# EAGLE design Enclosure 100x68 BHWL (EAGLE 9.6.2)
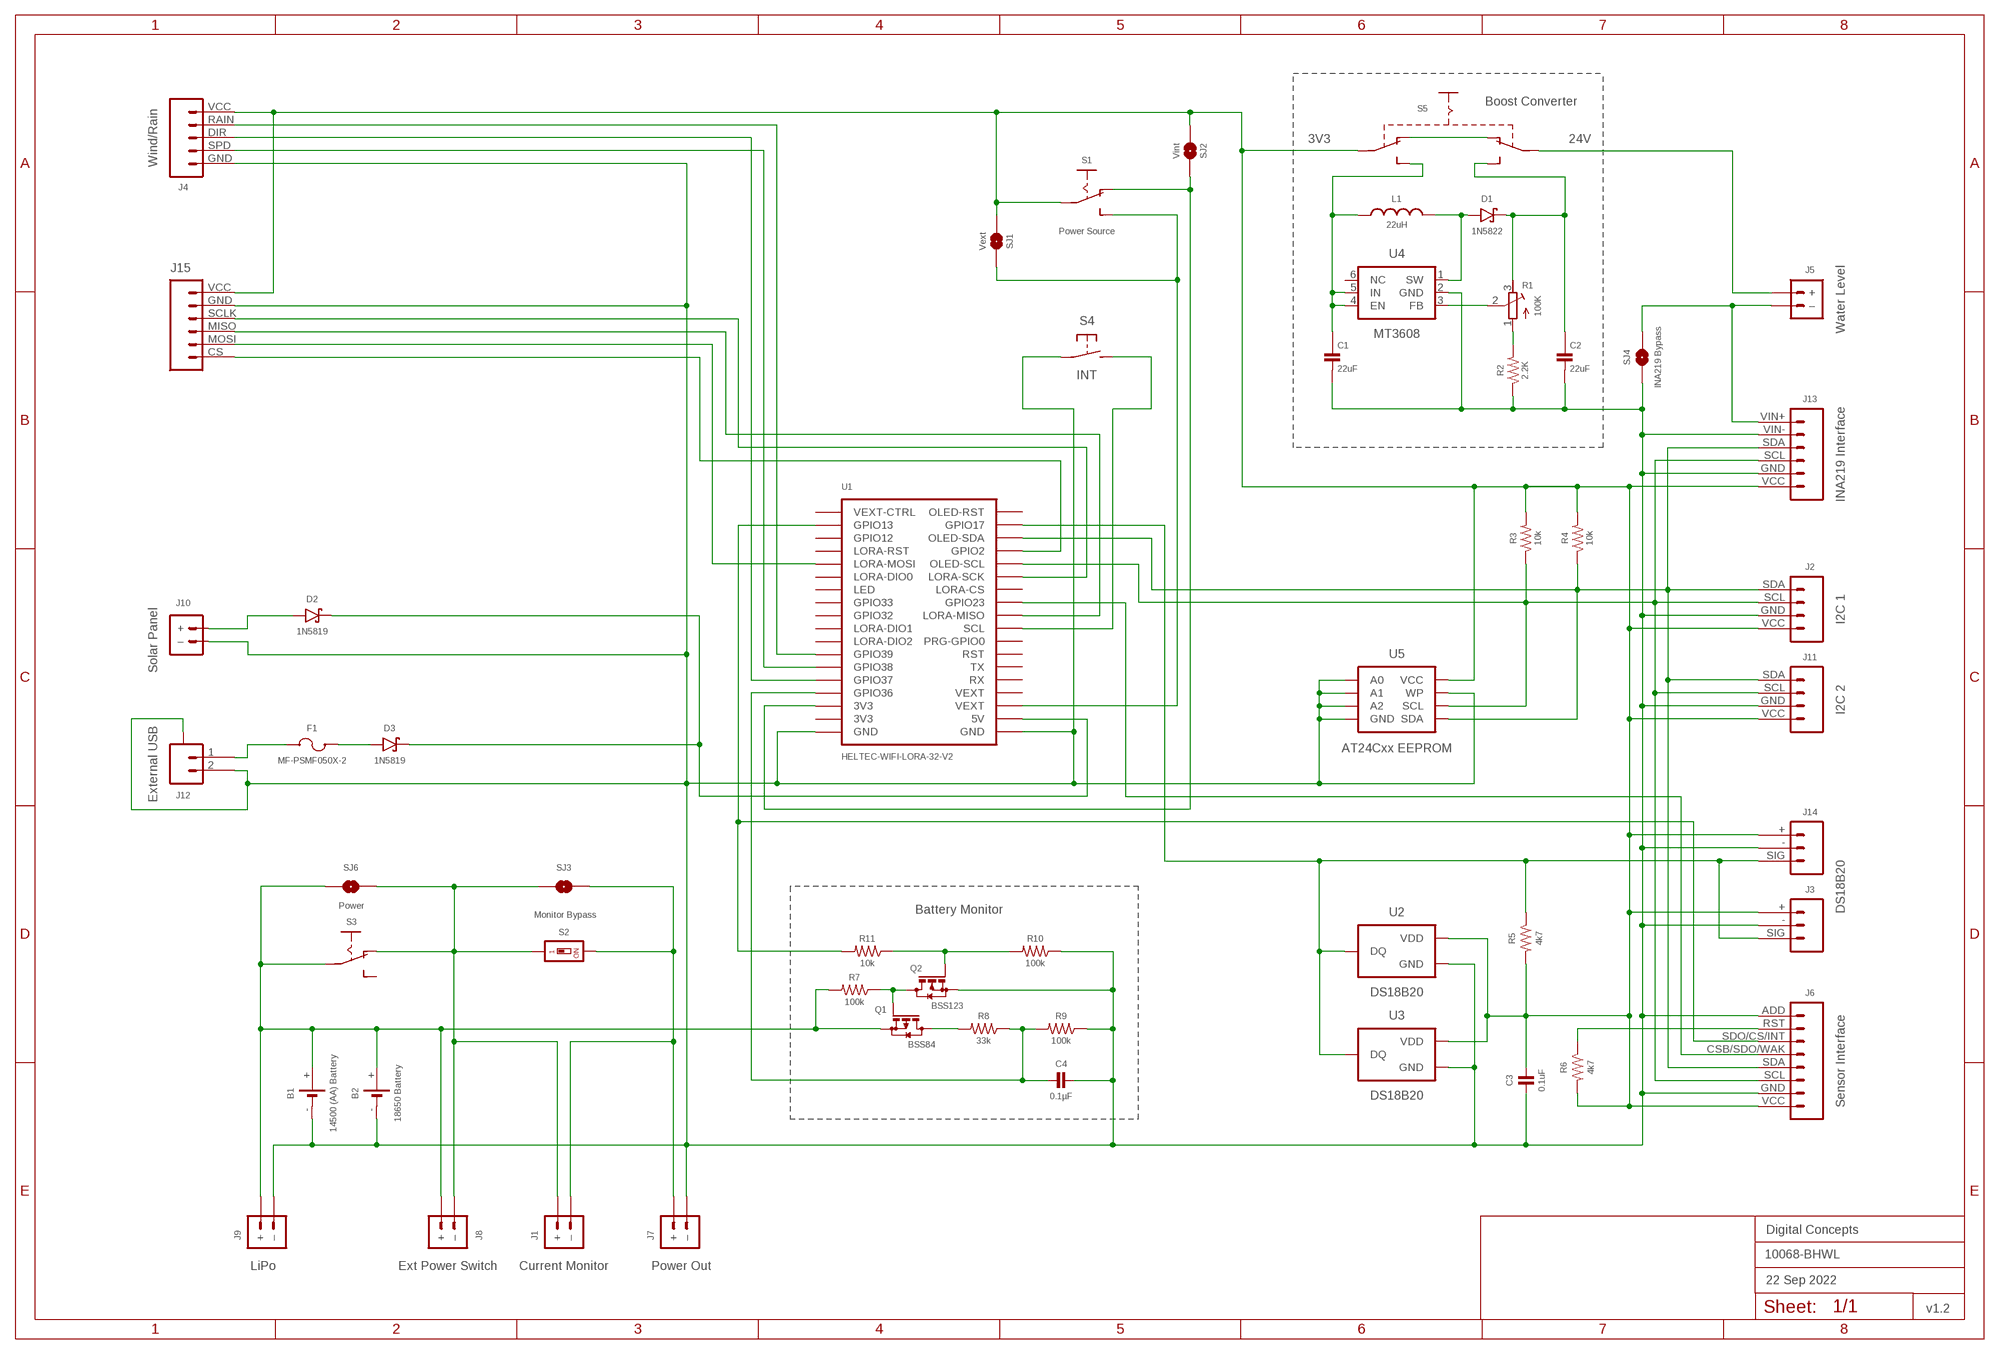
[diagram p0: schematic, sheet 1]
FRAME2 (A3L-LOC): DATE: 22 Sep 2022; OWNER: Digital Concepts; TITLE: 10068-BHWL; VERSION: v1.2

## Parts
B1  14500 (AA) Battery  BATTERY-HOLDER-14500(AA)  [BATTERY-14500]
B2  18650 Battery  BATTERY-HOLDER-18650  [BATTERY-18650]
C1  22uF  CAPACITOR-1206  [C1206]
C2  22uF  CAPACITOR-1206  [C1206]
C3  0.1uF  CAPACITOR-0805  [C0805]
C4  0.1µF  CAPACITOR-0805  [C0805]
D1  1N5822  DIODE-SCHOTTKY-1N5822  [DIODE_SMB]
D2  1N5819  1N5819-SOD-123  [SOD-123]
D3  1N5819  1N5819-SOD-123  [SOD-123]
F1  MF-PSMF050X-2  [F0805]
J1  Current Monitor  JST-PH2.0-2-HORIZONTALJST-PTH-2  [JST-PH2.0-2-HORIZONTAL]
J2  I2C 1  JST-PH2.0-4-VERTICAL-I2C  [JST-PH2.0-4-VERTICAL-I2C]
J3  DS18B20  JST-PH2.0-3-VERTICAL-DS18B20  [JST-PH2.0-3-VERTICAL-SIG]
J4  Wind/Rain  JST-PH2.0-5-DUAL-WEATHER  [JST-PH2.0-5-DUAL-WEATHER]
J5  Water Level  JST-PH2.0-2-DUAL-POWERJST-PTH-2  [JST-PH2.0-2-DUAL-POWER]
J6  Sensor Interface  HEADER-1X8-SENSOR  [CONN_08-SENSOR]
J7  Power Out  JST-GH1.25-2-HORIZONTAL-POWER  [JST-GH1.25-2-HORIZONTAL]
J8  Ext Power Switch  JST-PH2.0-2-DUAL-POWERJST-PTH-2  [JST-PH2.0-2-DUAL-POWER]
J9  LiPo  JST-PH2.0-2-HORIZONTAL-POWERJST-PTH-2  [JST-PH2.0-2-HORIZONTAL-POWER]
J10  Solar Panel  JST-PH2.0-2-VERTICAL  [JST-PH2.0-2-VERTICAL=POWER]
J11  I2C 2  JST-PH2.0-I2C-MALE-HORIZONTAL  [JST-PH2.0-4-HORIZONTAL]
J12  External USB  JST-SH1.0-2-SMD-HORIZONTAL  [JST-SH1.0-2-HORIZONTAL]
J13  INA219 Interface  INA219-I2C-MODULE  [CONN_06-INA219]
J14  JST-PH2.0-3-HORIZONTAL-DS18B20  [JST-PH2.0-DS18B20-HORIZONTAL]
J15  JST-PH2.0-6-HORIZONTAL-SPI  [JST-PH2.0-6-HORIZONTAL-SPI]
L1  22uH  INDUCTOR-CDRH104R/6D28L5038P  [CDRH104R+6D28]
Q1  BSS84  [SOT23-3]
Q2  BSS123  MOSFET-BSS123  [SOT23-3]
R1  100K  RESISTOR-TRIMM-BAOTER-HORIZONTAL  [RTRIM64P]
R2  2.2K  RESISTORR0805  [R0805]
R3  10k  RESISTORR0805  [R0805]
R4  10k  RESISTORR0805  [R0805]
R5  4k7  RESISTORR0805  [R0805]
R6  4k7  RESISTORR0805  [R0805]
R7  100k  RESISTORR0805  [R0805]
R8  33k  RESISTORR0805  [R0805]
R9  100k  RESISTORR0805  [R0805]
R10  100k  RESISTORR0805  [R0805]
R11  10k  RESISTORR0805  [R0805]
S1  Power Source  SWITCH-SLIDE-SPDT-SMT  [SWITCH-SPDT-SMT]
S2  Monitor Bypass  SWITCH-DIP-SWS001  [SMD-001]
S3  Power  SWITCH-SLIDE-SPDT-PTH  [SWITCH-SPDT-PTH]
S4  INT  SWITCH-MOMENTARY-2-PIN  [SWITCH-2-PAD]
S5  SWITCH-SLIDE-DPDT-PTH-S  [SWITCH-DPDT-PTH]
SJ1  Vext  SJ  [SJ]
SJ2  Vint  SJ-V-2  [SJ-VIA-2]
SJ3  Monitor  SJ  [SJ]
SJ4  INA219 Bypass  SJ  [SJ]
SJ6  Power  SJ  [SJ]
U1  HELTEC-WIFI-LORA-32-V2  [HELTEC-WIFI-LORA-32-V2]
U2  DS18B20  THERMOMETER-DS18B20  [TO-92]
U3  DS18B20  THERMOMETER-DS18B20  [TO-92]
U4  MT3608  [SOT-23-6]
U5  AT24Cxx EEPROM  AT24CXX-EEPROM  [SOP-8]

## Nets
GND: B1.- B2.- C1.2 C2.2 C3.2 C4.2 J2.GND J3.- J4.GND J6.ADD J6.GND J7.-(–) J9.-(–) J10.-(–) J11.GND J12.2 J12.A@1(A) J12.A@2(A) J13.GND J13.VIN- J14.- J15.GND Q2.2(S) R2.1 R9.1 R10.1 S4.P$1(P) SJ4.1 U1.GND@1(GND) U1.GND@36(GND) U2.1(GND) U3.1(GND) U4.2(GND) U5.P$1(A0) U5.P$2(A1) U5.P$3(A2) U5.P$4(GND) U5.P$7(WP)
N$1: D2.A J10.+
N$2: J4.RAIN U1.GPIO39
N$3: J6.CSB/SDO/WAK U1.GPIO23
N$4: J2.SCL J6.SCL J11.SCL J13.SCL R3.1 U1.GPIO15(OLED-SCL) U5.P$6(SCL)
N$5: D2.C D3.C U1.5V
N$6: D1.A L1.1 U4.1(SW)
N$7: Q1.3(D) R8.2
N$8: J1.2(–) J7.+ S2.2 SJ3.1
N$9: J6.RST R6.1
N$10: J4.DIR U1.GPIO37
N$11: J2.SDA J6.SDA J11.SDA J13.SDA R4.1 U1.GPIO4(OLED-SDA) U5.P$5(SDA)
N$12: J4.SPD U1.GPIO38
N$13: S1.3(S) SJ1.1 U1.VEXT@3(VEXT)
N$14: F1.2 J12.1
N$15: J5.-(–) J13.VIN+ SJ4.2
N$16: D3.A F1.1
N$17: S4.P$2(S) U1.GPIO22(SCL)
N$18: C4.1 R8.1 R9.2 U1.GPIO36
N$19: S1.1(O) SJ2.1 U1.3V3@34(3V3)
N$20: J5.+ S5.P$2(P1)
N$21: J1.1(+) J8.-(–) S2.1 S3.1(O) SJ3.2 SJ6.1
N$22: R1.2(S) U4.3(FB)
N$23: R1.1(A) R2.2
N$24: J3.SIG J14.SIG R5.1 U1.GPIO17 U2.2(DQ) U3.2(DQ)
N$25: C1.1 L1.2 S5.P$6(S2) U4.4(EN) U4.5(IN)
N$26: S5.P$1(O1) S5.P$4(O2)
N$27: J15.SCLK U1.GPIO5(LORA-SCK)
N$28: C2.1 D1.C R1.3(E) S5.P$3(S1)
N$29: J15.MOSI U1.GPIO27(LORA-MOSI)
N$30: B1.+ B2.+ J8.+ J9.+ Q1.2(S) R7.2 S3.2(P) SJ6.2
N$31: J15.MISO U1.GPIO19(LORA-MISO)
N$32: J6.SDO/CS/INT R11.2 U1.GPIO13
N$33: J15.CS U1.GPIO2
N$35: Q1.1(G) Q2.3(D) R7.1
N$37: Q2.1(G) R10.2 R11.1
VEXT: C3.1 J2.VCC J3.+ J4.VCC J6.VCC J11.VCC J13.VCC J14.+ J15.VCC R3.2 R4.2 R5.2 R6.2 S1.2(P) S5.P$5(P2) SJ1.2 SJ2.2 SJ2.2@V U2.3(VDD) U3.3(VDD) U5.P$8(VCC)
Unconnected: S3.3(S) U1.3V3@35(3V3) U1.GPIO0(PRG-GPIO0) U1.GPIO12 U1.GPIO14(LORA-RST) U1.GPIO16(OLED-RST) U1.GPIO18(LORA-CS) U1.GPIO21(VEXT-CTRL) U1.GPIO25(LED) U1.GPIO26(LORA-DIO0) U1.GPIO32 U1.GPIO33 U1.GPIO34(LORA-DIO2) U1.GPIO35(LORA-DIO1) U1.RST U1.RX U1.TX U1.VEXT@4(VEXT) U4.6(NC)

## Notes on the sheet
- Boost Converter
- 3V3 | 24V
- Battery Monitor

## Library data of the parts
B1 = digitalconcepts:BATTERY-HOLDER-14500(AA): 14500 (AA) battery holder
B2 = digitalconcepts:BATTERY-HOLDER-18650: 18650 Battery Holder
C1 C2 = digitalconcepts:CAPACITOR-1206: 1206 Capacitor
C3 C4 = digitalconcepts:CAPACITOR-0805: 0805 Capacitor
D1 = digitalconcepts:DIODE-SCHOTTKY-1N5822: 1N5822 Schottky Diode SMB
D2 D3 = digitalconcepts:1N5819-SOD-123: 1N5819 Schottky Diode SOD-123
F1 = digitalconcepts:MF-PSMF050X-2: PTC Resettable Fuse
J1 = digitalconcepts:JST-PH2.0-2-HORIZONTAL: PH2.0 2P Right Angle PCB Connector; PROD_ID: CONN-09863; SKU: PRT-09914
J2 = digitalconcepts:JST-PH2.0-4-VERTICAL-I2C: PH2.0 4P I2C Vertical Connector
J3 = digitalconcepts:JST-PH2.0-3-VERTICAL-DS18B20: DS18B20 PH2.0 Vertical PCB Connector
J4 = digitalconcepts:JST-PH2.0-5-DUAL-WEATHER: PH2.0 5P Dual Connector
J5 J8 = digitalconcepts:JST-PH2.0-2-DUAL-POWER: JST PH2.0 2P PTH Dual-Side Connector (Power); PROD_ID: CONN-09863; SKU: PRT-09914
J6 = digitalconcepts:HEADER-1X8-SENSOR: IoT Sensors 1x8 Pin Header for 'Sandwich' IoT Sensors
J7 = digitalconcepts:JST-GH1.25-2-HORIZONTAL-POWER: JST GH1.25 2P PTH Connector (Power)
J9 = digitalconcepts:JST-PH2.0-2-HORIZONTAL-POWER: PH2.0 2P Right Angle PCB Connector; PROD_ID: CONN-09863; SKU: PRT-09914
J10 = digitalconcepts:JST-PH2.0-2-VERTICAL: PH2.0 2P PCB Connector
J11 = digitalconcepts:JST-PH2.0-I2C-MALE-HORIZONTAL: PH2.0 4P (I2C) Right Angle PCB Connector
J12 = digitalconcepts:JST-SH1.0-2-SMD-HORIZONTAL: JST SH1.0 2P SMD Horizontal Connector
J13 = digitalconcepts:INA219-I2C-MODULE: INA219 I2C Module
J14 = digitalconcepts:JST-PH2.0-3-HORIZONTAL-DS18B20: DS18B20 PH2.0 Right Angle PCB Connector
J15 = digitalconcepts:JST-PH2.0-6-HORIZONTAL-SPI: PH2.0 6P Horizontal Connector—SPI
L1 = digitalconcepts:INDUCTOR-CDRH104R/6D28: Inductor; SPICEPREFIX: L
Q1 = digitalconcepts:BSS84: P-CHANNEL MOS FET
Q2 = digitalconcepts:MOSFET-BSS123: N-CHANNEL MOS FET
R1 = digitalconcepts:RESISTOR-TRIMM-BAOTER-HORIZONTAL: Trimm Resistor - Horizontal BAOTER
R2-R11 = digitalconcepts:RESISTOR: Resistor; SPICEPREFIX: R
S1 = digitalconcepts:SWITCH-SLIDE-SPDT-SMT: Mini Sliding Switch SPDT SMT
S2 = digitalconcepts:SWITCH-DIP-SWS001: SMD Dip Switch 1 pol.
S3 = digitalconcepts:SWITCH-SLIDE-SPDT-PTH: Mini Sliding Switch SPDT PTH
S4 = digitalconcepts:SWITCH-MOMENTARY-2-PIN: 2 Pin Momentary Switch
S5 = digitalconcepts:SWITCH-SLIDE-DPDT-PTH-S: Switch DPDT PTH-S
SJ1 SJ3 SJ4 SJ6 = digitalconcepts:SJ: Solder Jumper
SJ2 = digitalconcepts:SJ-V-2: Solder Jumper with Pad Vias
U1 = digitalconcepts:HELTEC-WIFI-LORA-32-V2: Heltec WiFi LoRa 32 Development Board V2
U2 U3 = digitalconcepts:THERMOMETER-DS18B20: Digital Thermometer -55C-125C TO92-3; AVAILABILITY: Bad; DESCRIPTION: Temperature Sensor Digital, Local -55°C ~ 125°C 12 b 8-uMAX; MF: Maxim Integrated; MP: DS18B20; PACKAGE: TO-92 Maxim Integrated; PRICE: None
U4 = digitalconcepts:MT3608: MT3608 DC-DC Step-Up Voltage Converter
U5 = digitalconcepts:AT24CXX-EEPROM: AT24Cxx EEPROM SOP-8

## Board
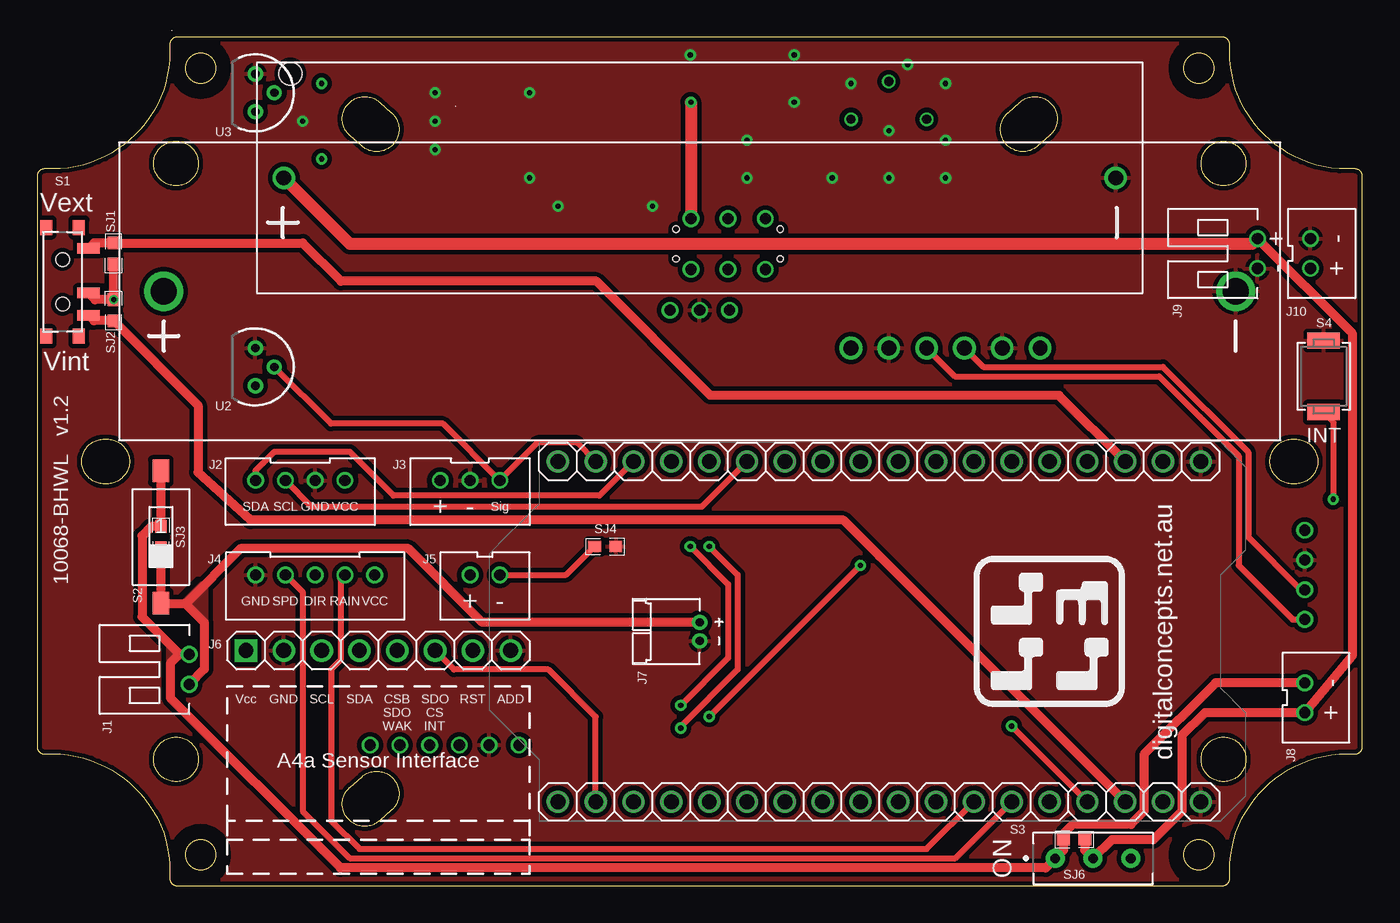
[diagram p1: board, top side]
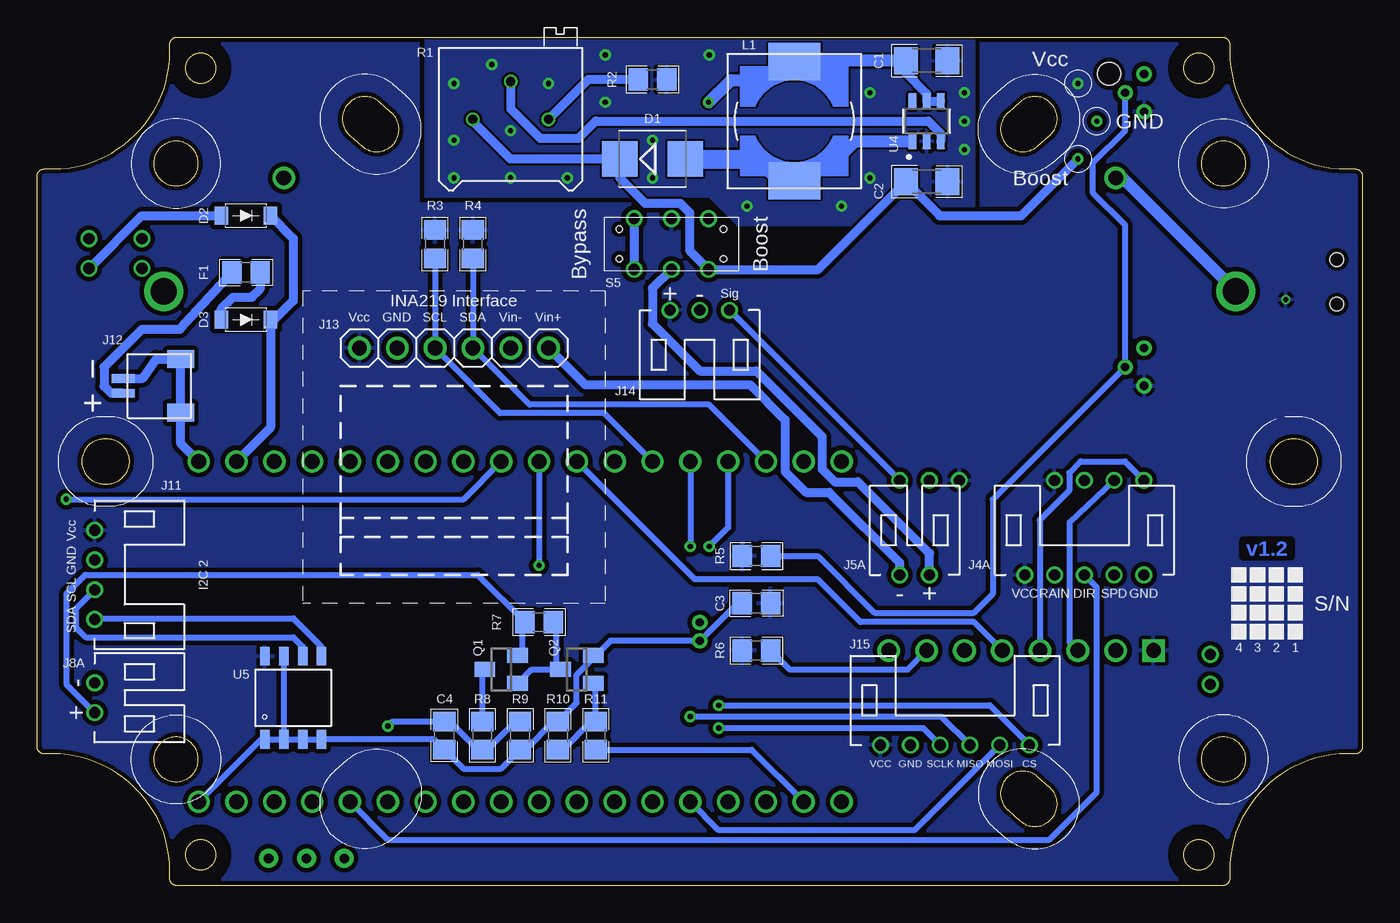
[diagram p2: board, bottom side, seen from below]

Size 89 x 57 mm. Coordinates in mm from the lower left corner, seen from the top.
Outline: 1134 segments
Outline: circle at 10.97,2.08 radius 1.02
Outline: circle at 10.97,54.92 radius 1.02
Outline: circle at 78.03,54.92 radius 1.02
Outline: circle at 78.03,2.08 radius 1.02
Copper layers (1*16): Top 0.035mm / dielectric 1.5mm / Bottom 0.035mm
Design rules "default *": minimum track width 6mil, minimum drill 0.35mm, track to track 6mil, track to pad 6mil, pad to pad 6mil, via to via 6mil, smd to smd 6mil, copper to edge 6mil, drill to drill 6mil, minimum pad ring 1mil, minimum via ring 8mil, stop-mask expansion 4mil, vias tented up to drill 0mil, thermal gap 10mil

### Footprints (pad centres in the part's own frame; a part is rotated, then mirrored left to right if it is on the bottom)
BATTERY-14500 = drill 1: + -27.94,0; - 27.94,0 | hole 1.524: -27.5,7
BATTERY-18650 = drill 1.75: + -36,0; - 36,0
C1206 = smd 1.6 x 1.8: 1 -1.4,0; 2 1.4,0
C0805 = smd 1.3 x 1.5: 1 -0.95,0; 2 0.95,0
DIODE_SMB = smd 2.4 x 2.4: A 2.2,0; C -2.2,0
SOD-123 = smd 0.91 x 1.22: A -1.65,0; C 1.65,0
F0805 = smd 1.3 x 1.5: 1 -0.95,0; 2 0.95,0
JST-PH2.0-2-HORIZONTAL = drill 0.75: 1 1,0; 2 -1,0
JST-PH2.0-4-VERTICAL-I2C = drill 0.75: GND 1,0; SCL -1,0; SDA -3,0; VCC 3,0
JST-PH2.0-3-VERTICAL-SIG = drill 0.75: + -2,0; - 0,0; SIG 2,0
JST-PH2.0-5-DUAL-WEATHER = drill 0.75: DIR 0,0; GND 4,0; RAIN -2,0; SPD 2,0; VCC -4,0
JST-PH2.0-2-DUAL-POWER = drill 0.75: + 1,0; - -1,0
CONN_08-SENSOR = drill 1 pad 1.524: ADD 17.78,0; CSB/SDO/WAK 10.16,0; GND 2.54,0; RST 15.24,0; SCL 5.08,0; SDA 7.62,0; SDO/CS/INT 12.7,0 | drill 1 pad 1.524 square: VCC 0,0
JST-GH1.25-2-HORIZONTAL = drill 0.55 pad 1.016: + -0.625,0; - 0.625,0
JST-PH2.0-2-HORIZONTAL-POWER = drill 0.75: + 1,0; - -1,0
JST-PH2.0-2-VERTICAL=POWER = drill 0.75: + -1,0; - 1,0
JST-PH2.0-4-HORIZONTAL = drill 0.75: GND -1,0; SCL 1,0; SDA 3,0; VCC -3,0
JST-SH1.0-2-HORIZONTAL = smd 0.6 x 1.55: 1 -0.5,2.54; 2 0.5,2.54 | smd 1.2 x 1.8: A@1 -1.8,-1.335; A@2 1.8,-1.335
CONN_06-INA219 = drill 1 pad 1.524: GND 2.54,0; SCL 5.08,0; SDA 7.62,0; VCC 0,0; VIN+ 12.7,0; VIN- 10.16,0
JST-PH2.0-DS18B20-HORIZONTAL = drill 0.75: + 2,0; - 0,0; SIG -2,0
JST-PH2.0-6-HORIZONTAL-SPI = drill 0.75: CS 5,0; GND -3,0; MISO 1,0; MOSI 3,0; SCLK -1,0; VCC -5,0
CDRH104R+6D28 = smd 2.5 x 3.5: 1 -4,0; 2 4,0
SOT23-3 = smd 1 x 1.4: 1 -0.95,-1.1; 2 0.95,-1.1; 3 0,1.1
RTRIM64P = drill 0.61: 1 0,-2.54; 2 2.54,0; 3 0,2.54
R0805 = smd 1.3 x 1.5: 1 -0.95,0; 2 0.95,0
SWITCH-SPDT-SMT = smd 0.7 x 1.5: 1 2.25,1.75; 2 0.75,1.75; 3 -2.25,1.75 | smd 1 x 0.8: GND@1 3.65,-1.1; GND@2 3.65,1.1; GND@3 -3.65,1.1; GND@4 -3.65,-1.1 | hole 0.9: -1.5,0; 1.5,0
SMD-001 = smd 1.1 x 1.5: 1 0,-4.45; 2 0,4.45
SWITCH-SPDT-PTH = drill 0.65 pad 1.27: 1 -2.54,0; 2 0,0; 3 2.54,0
SWITCH-2-PAD = smd 1.067 x 2.184: P$1 -2.4,0; P$2 2.4,0
SWITCH-DPDT-PTH = drill 0.75: P$1 -1.7,2.5; P$2 -1.7,0; P$3 -1.7,-2.5; P$4 1.7,2.5; P$5 1.7,0; P$6 1.7,-2.5 | hole 0.42: 1,3.5; -1,3.5; 1,-3.5; -1,-3.5
SJ = smd 0.864 x 0.762: 1 -0.711,0; 2 0.711,0
SJ-VIA-2 = smd 0.864 x 0.762: 1 -0.711,0; 2 0.711,0 | drill 0.35 pad 0.61: 2@V 0.711,0
HELTEC-WIFI-LORA-32-V2 = drill 1: 3V3@34 -22.86,5.08; 3V3@35 -22.86,2.54; 5V 0,2.54; GND@1 0,0; GND@36 -22.86,0; GPIO0 0,17.78; GPIO2 0,35.56; GPIO4 0,38.1; GPIO5 0,33.02; GPIO12 -22.86,38.1; GPIO13 -22.86,40.64; GPIO14 -22.86,35.56; GPIO15 0,30.48; GPIO16 0,43.18; GPIO17 0,40.64; GPIO18 0,27.94; GPIO19 0,22.86; GPIO21 -22.86,43.18; GPIO22 0,20.32; GPIO23 0,25.4; GPIO25 -22.86,27.94; GPIO26 -22.86,30.48; GPIO27 -22.86,33.02; GPIO32 -22.86,22.86; GPIO33 -22.86,25.4; GPIO34 -22.86,17.78; GPIO35 -22.86,20.32; GPIO36 -22.86,7.62; GPIO37 -22.86,10.16; GPIO38 -22.86,12.7; GPIO39 -22.86,15.24; RST 0,15.24; RX 0,10.16; TX 0,12.7; VEXT@3 0,5.08; VEXT@4 0,7.62
TO-92 = drill 0.55 pad 1.016: 1 -1.27,0; 2 0,1.27; 3 1.27,0
SOT-23-6 = smd 1.1 x 0.6: 1 -1.35,0.95; 2 -1.35,0; 3 -1.35,-0.95; 4 1.35,-0.95; 5 1.35,0; 6 1.35,0.95
SOP-8 = smd 0.635 x 1.27: P$1 -1.905,-2.794; P$2 -0.635,-2.794; P$3 0.635,-2.794; P$4 1.905,-2.794; P$5 1.905,2.794; P$6 0.635,2.794; P$7 -0.635,2.794; P$8 -1.905,2.794

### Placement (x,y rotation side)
B1  44.5,47.55 0 top
B2  44.5,39.93 0 top
C1  29.26,55.42 0 bottom
C2  29.26,47.3 0 bottom
C3  40.69,18.97 180 bottom
C4  61.64,10.08 270 bottom
D1  47.67,48.82 0 bottom
D2  74.98,45.01 0 bottom
D3  74.98,38.02 0 bottom
F1  74.98,41.2 180 bottom
J1  10.21,14.53 90 top
J2  17.67,27.23 0 top
J3  29.07,27.23 0 top
J4  18.67,20.88 0 bottom
J5  30.07,20.88 0 bottom
J6  14.02,15.8 0 top
J7  44.5,17.07 270 top
J8  85.14,12.62 270 bottom
J9  81.96,42.47 90 top
J10  85.52,42.47 90 top
J11  85.14,20.88 270 bottom
J12  80.69,33.58 90 bottom
J13  67.36,36.12 0 bottom
J14  44.5,38.66 180 bottom
J15  27.35,9.45 0 bottom
L1  38.15,51.36 90 bottom
Q1  57.83,14.53 90 bottom
Q2  52.75,14.53 90 bottom
R1  57.2,51.49 90 bottom
R2  47.67,54.15 180 bottom
R3  62.28,43.1 90 bottom
R4  59.74,43.1 90 bottom
R5  40.69,22.15 180 bottom
R6  40.69,15.8 180 bottom
R7  55.29,17.7 180 bottom
R8  59.1,10.08 90 bottom
R9  56.56,10.08 90 bottom
R10  54.02,10.08 270 bottom
R11  51.48,10.08 270 bottom
S1  1.7,40.56 270 top
S2  8.3,23.42 180 top
S3  70.92,1.83 0 top
S4  86.41,34.21 270 top
S5  46.4,43.1 90 bottom
SJ1  5.13,42.47 270 top
SJ2  5.13,38.66 90 top
SJ3  8.3,23.42 90 top
SJ4  38.15,22.78 180 top
SJ6  69.65,3.1 0 top
U1  78.15,28.5 90 top
U2  14.65,34.85 270 top
U3  14.65,53.26 270 top
U4  29.26,51.36 90 bottom
U5  71.8,12.62 0 bottom

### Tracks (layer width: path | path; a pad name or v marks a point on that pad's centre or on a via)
$X
  cutout Bottom: 10.97,56.95 arc180 10.97,52.88 arc180
$X1
  cutout Bottom: 78.03,56.95 arc180 78.03,52.88 arc180
$X2
  cutout Top: 78.03,4.12 arc180 78.03,0.05 arc180
$X3
  cutout Top: 10.97,4.12 arc180 10.97,0.05 arc180
$X4
  cutout Top: 10.97,56.95 arc180 10.97,52.88 arc180
$X5
  cutout Top: 78.03,56.95 arc180 78.03,52.88 arc180
$X6
  cutout Bottom: 78.03,4.12 arc180 78.03,0.05 arc180
$X7
  cutout Bottom: 10.97,4.12 arc180 10.97,0.05 arc180
GND  (via drill 0.35)
  Bottom 0.406: U5.P$7 U5.P$2 | U5.P$2 U5.P$1 73.96,9.83 U1.GND@36 | U5.P$2 U5.P$3 U5.P$4 62.34,9.83 C4.2 60.37,7.86 57.83,7.86 R9.1 56.21,9.13 54.31,11.03 R10.1 52.76,12.3 52.76,14.18 51.65,15.28 | 51.65,15.28 Q2.2 | C3.2 41.97,18.97 J7.- 50.49,16.44 51.65,15.28
  Bottom 0.61: J12.2 81.93,34.08 81,35.38 J12.A@2 J12.A@1 79.36,29.7 U1.GND@1
  other vias: 26.72,53.26 50.85,55.8 50.85,52.63 47.67,50.09 47.67,47.55 53.39,47.55 57.2,47.55 57.2,50.72 61.01,47.55 61.01,50.09 58.47,55.17 26.72,51.36 54.66,53.9 61.01,53.9 43.86,55.8 33.07,53.26 33.07,47.55 26.72,49.45 17.83,51.36 34.97,45.64 41.32,45.64
  pour Top (isolate 0.305, rank 2): -1.65,58.87 -1.65,-1.92 90.59,-1.92 90.59,58.87
  pour Bottom: 26.08,57.07 26.08,45.64 33.07,45.64 34.34,44.37 41.96,44.37 43.86,46.28 62.91,46.28 62.91,57.07
N$1
  Bottom 0.61: J10.+ 81.98,45.01 D2.A
N$2
  Top 0.406: J4.RAIN 20.37,20.58 20.37,15.16 19.73,14.53 19.73,4.37 21.64,2.46 59.74,2.46 U1.GPIO39
N$3
  Bottom 0.406: J6.CSB/SDO/WAK 26.08,17.7 33.7,17.7 36.57,20.57 44.83,20.57 U1.GPIO23
N$4
  Top 0.406: J13.SCL 63.55,34.85 75.61,34.85 81.33,29.13 81.33,23.42 84.87,19.88 J11.SCL | U1.GPIO15 44.63,25.45 18.45,25.45 J2.SCL
  Bottom 0.406: J2.SCL 19.66,24.41 19.66,16.36 J6.SCL | U5.P$6 71.17,16.05 71.8,16.69 85.76,16.69 86.41,17.34 86.41,18.61 J11.SCL | R3.1 J13.SCL 57.91,31.75 50.93,31.75 U1.GPIO15
N$5
  Bottom 0.61: D2.C 71.8,43.48 71.8,39.29 73.07,38.02 D3.C 73.33,30.78 U1.5V
N$6
  Bottom 0.152: U4.1 30.4,50.01
  Bottom 0.813: 40.68,48.82 38.96,47.11 L1.1 36.84,48.27 35.79,48.27 34.05,50.01 30.4,50.01
  Bottom 1.27: D1.A 40.68,48.82
N$7
  Bottom 0.406: Q1.3 59.1,14.36 R8.2
N$8
  Top 0.61: J1.2 11.23,14.55 11.23,17.67 9.96,18.94 | 9.96,18.94 9.93,18.97 S2.2 SJ3.1 | 9.96,18.94 13.66,22.65 24.94,22.65 29.89,17.69 J7.+
  pour Top (no thermals): 9.93,18.98 11.23,17.7 11.23,20.26
N$9
  Bottom 0.406: J6.RST 30.53,14.53 38.47,14.53 R6.1
N$10
  Bottom 0.406: U1.GPIO37 65.45,3.1 21,3.1 17.83,6.27 17.83,20.04 J4.DIR
N$11
  Top 0.406: J13.SDA 61.64,34.21 75.36,34.21 80.69,28.88 80.69,21.51 84.33,17.88 J11.SDA | U1.GPIO4 37.77,26.21 23.93,26.21 21,29.13 15.92,29.13 14.67,27.88 J2.SDA
  Bottom 0.406: J6.SDA 21.66,15.82 21.66,24.56 19.68,26.54 19.68,27.73 18.92,28.5 15.94,28.5 J2.SDA | J11.SDA 85.06,17.96 71.8,17.96 69.9,16.05 U5.P$5 | R4.1 J13.SDA 55.93,32.31 43.86,32.31 U1.GPIO4
N$12
  Top 0.406: J4.SPD 17.83,19.72 17.83,5 20.98,1.85 61.67,1.85 U1.GPIO38
N$13
  Top 0.61: S1.3 3.82,43.18 SJ1.1 17.83,43.18 20.41,40.6 37.55,40.6 45.21,32.94 68.63,32.94 U1.VEXT@3
N$14
  Bottom 0.61: J12.1 84.02,33.08 84.5,33.56 84.5,34.85 81.96,37.39 79.42,37.39 F1.2
N$15
  Top 0.406: SJ4.2 35.53,20.88 J5.-
  Bottom 0.61: J5.- 31.07,21.69 35.8,26.42 37.35,26.42 38.77,27.84 38.77,31.29 41.13,33.66 52.2,33.66 J13.VIN+
N$16
  Bottom 0.61: D3.A 76.63,38.76 75.85,39.53 74.58,39.53 74.03,40.09 F1.1
N$17  (via drill 0.35)
  Top 0.406: S4.P$2 87.04,31.18 v87.04,25.96
  Bottom 0.406: v87.04,25.96 60.37,25.96 U1.GPIO22
N$18  (via drill 0.35)
  Top 0.406: U1.GPIO36 v65.45,10.72
  Bottom 0.406: R9.2 56.87,11.03 58.77,9.13 R8.1 59.38,9.13 61.29,11.03 C4.1 65.14,11.03 v65.45,10.72
N$19
  Top 0.61: S1.1 3.82,37.95 SJ2.1 10.81,32.27 10.81,27.77 14.34,24.56 54.15,24.56 56.56,22.15 U1.3V3@34
N$20
  Bottom 0.61: S5.P$2 47.67,40.13 47.67,37.75 44.5,34.58 40.69,34.58 36.28,30.17 36.28,27.98 35.43,27.13 33.88,27.13 29.07,22.32 J5.+
N$21
  Top 0.61: S2.1 SJ3.2 7.67,24.13 7.03,23.5 7.03,18.07 9.57,15.53 J1.1 9.55,15.53 8.94,14.92 8.94,12.62 20.37,1.19 67.74,1.19 S3.1 68.93,2.39 SJ6.1 68.93,3.48 69.57,4.12 73.46,4.12 74.34,5 74.34,8.81 79.15,13.62 J8.-
  pour Top (no thermals): 9.55,15.55 8.94,16.16 8.94,14.94
N$22
  Bottom 0.61: R1.2 57.2,52.2 55.22,50.22 52.63,50.22 51.48,51.36 29.16,51.36 28.31,50.51 U4.3
N$23
  Bottom 0.61: R2.2 51.99,54.15 R1.1
N$24
  Top 0.406: U2.2 19.73,31.04 27.26,31.04 J3.SIG 33.61,29.77 36.24,29.77 U1.GPIO17
  Bottom 0.406: J14.SIG J3.SIG | R5.1 36.56,22.15 32.75,18.34 26.08,18.34 24.81,19.61 24.81,25.96 U2.2 15.92,44.37 18.08,46.53 18.08,48.57 15.92,50.72 U3.2
N$25  (via drill 0.35)
  Top 0.813: v43.9,52.63 S5.P$6
  Bottom 0.61: C1.1 30.66,54.61 29.26,53.21 U4.5 U4.4
  Bottom 0.813: C1.1 38.04,55.42 L1.2 38.99,55.36 39.98,54.12 42.41,54.12 v43.9,52.63
N$26
  Bottom 0.61: S5.P$4 S5.P$1
N$27  (via drill 0.35)
  Top 0.406: v45.13,22.78 47.04,20.88 47.04,14.53 43.23,10.72 v43.23,10.59
  Bottom 0.406: U1.GPIO5 v45.13,22.78 | v43.23,10.59 29.5,10.59 J15.SCLK
N$28  (via drill 0.35)
  Bottom 0.61: v19.1,48.82 22.91,45.01 28.37,45.01 C2.1 36.55,41.4 S5.P$3 45.17,42.67 45.17,45.21 45.81,45.85 48.17,45.85 49.87,47.55 D1.C 57.22,48.82 59.74,51.34 R1.3
N$29
  Bottom 0.406: J15.MOSI 30.07,3.73 43.23,3.73 U1.GPIO27
N$30
  Top 0.61: SJ6.2 70.36,2.39 S3.2 72.19,3.1 74.98,3.1 76.88,5 76.88,10.08 78.42,11.62 J8.+ 88.31,15.43 88.31,37.12 J9.+
  Top 0.813: J9.+ 81.6,43.1 21,43.1 B1.+
  Bottom 0.406: Q1.2 56.44,15.78 56.44,17.51 R7.2 59.42,20.88 85.77,20.88 87.04,19.61 87.04,13.53 J8.+
  Bottom 0.813: B1.+ 16.12,47.55 B2.+
N$31  (via drill 0.35)
  Top 0.406: v45.13,11.35 v55.29,21.51
  Bottom 0.406: U1.GPIO19 v55.29,21.51 | J15.MISO 28.26,11.35 v45.13,11.35
N$32
  Top 0.406: U1.GPIO13 37.51,11.35 34.34,14.53 27.99,14.53 J6.SDO/CS/INT
  Bottom 0.406: U1.GPIO13 41.01,9.13 R11.2
N$33  (via drill 0.35)
  Top 0.406: v43.86,22.78 46.4,20.24 46.4,15.29 v43.23,12.12
  Bottom 0.406: v43.86,22.78 42.59,24.05 U1.GPIO2 | J15.CS 25.02,12.12 v43.23,12.12
N$35
  Bottom 0.406: Q1.1 55.78,14.53 Q2.3 54.15,14.83 54.15,17.51 R7.1
N$37
  Bottom 0.406: R10.2 53.69,9.13 51.79,11.03 R11.1 51.48,13.41 Q2.1
VEXT  (via drill 0.35)
  Top 0.61: S1.2 3.89,39.37 SJ2.2@V SJ1.2
  other vias: 19.1,53.9
  pour Bottom (isolate 0.305, rank 2): -0.65,57.87 -0.65,-0.92 89.59,-0.92 89.59,57.87

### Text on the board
Bottom: v1.2
tPlace: 10068-BHWL v1.2 | digitalconcepts.net.au | Vcc | GND | SCL | SDA | RST | ADD | CSB / SDO / WAK | SDO / CS / INT
bPlace: Vin+ | Vin- | SDA | SCL | GND | Vcc | S/N | 1 | 2 | 3 | 4
tNames: Vext | Vint | A4a Sensor Interface | ON
bNames: Vcc | GND | Boost | Boost | Bypass | Vcc | GND | J4A | J5A | SCL | SDA | J8A
bValues: Wind/Rain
